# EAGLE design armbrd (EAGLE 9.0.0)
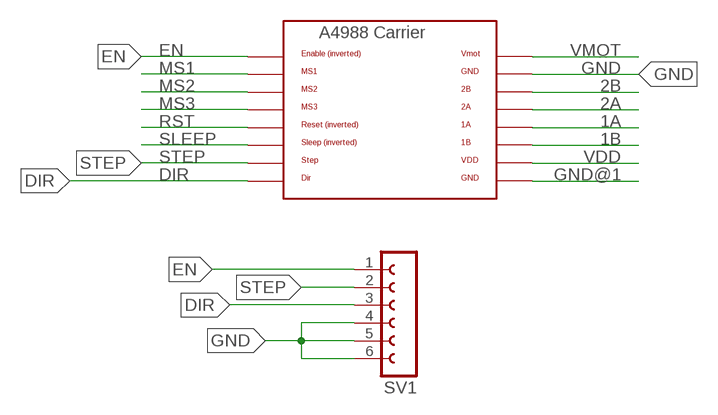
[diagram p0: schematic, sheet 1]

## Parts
SV1  FE06-1  [FE06]
U$1  A4988BREAKOUT  [A4988BREAKOUT]

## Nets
1A: U$1.1A
1B: U$1.1B
2A: U$1.2A
2B: U$1.2B
DIR: SV1.3 U$1.DIR
EN: SV1.1 U$1.EN
GND: SV1.4 SV1.5 SV1.6 U$1.GND
GND@1: U$1.GND@0(GND)
MS1: U$1.MS1
MS2: U$1.MS2
MS3: U$1.MS3
RST: U$1.RST
SLEEP: U$1.SLP(SLEEP)
STEP: SV1.2 U$1.STEP
VDD: U$1.VDD
VMOT: U$1.VMOT

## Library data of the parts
SV1 = con-lsta:FE06-1: FEMALE HEADER; OC_FARNELL: unknown; OC_NEWARK: unknown
U$1 = RepRapjr:A4988BREAKOUT

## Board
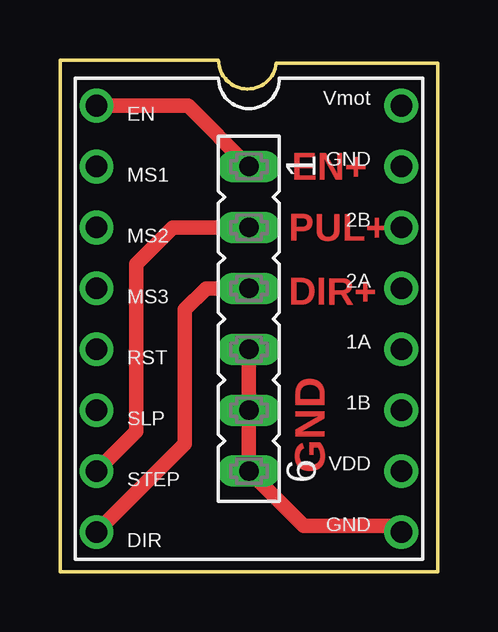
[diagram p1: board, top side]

Size 15.75 x 21.34 mm. Coordinates in mm from the lower left corner, seen from the top.
Outline: 0,21.34 6.6,21.34 arc174 9.02,21.21 15.75,21.21 15.75,0 0,0 0,21.34
Copper layers (1*16): Top 0.035mm / dielectric 1.5mm / Bottom 0.035mm
Design rules "default": minimum track width 6mil, minimum drill 0.35mm, track to track 6mil, track to pad 6mil, pad to pad 6mil, via to via 6mil, smd to smd 6mil, copper to edge 40mil, drill to drill 6mil, minimum pad ring 10mil, minimum via ring 8mil, stop-mask expansion 4mil, vias tented up to drill 0mil, thermal gap 10mil

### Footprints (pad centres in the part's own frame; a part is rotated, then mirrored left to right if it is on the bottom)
FE06 = drill 0.813 long: 1 -6.35,0; 2 -3.81,0; 3 -1.27,0; 4 1.27,0; 5 3.81,0; 6 6.35,0
A4988BREAKOUT = drill 0.9: 1A 8.89,1.27; 1B 11.43,1.27; 2A 6.35,1.27; 2B 3.81,1.27; DIR 16.51,-11.43; EN -1.27,-11.43; GND 16.51,1.27; GND@0 1.27,1.27; MS1 1.27,-11.43; MS2 3.81,-11.43; MS3 6.35,-11.43; RST 8.89,-11.43; SLP 11.43,-11.43; STEP 13.97,-11.43; VDD 13.97,1.27; VMOT -1.27,1.27

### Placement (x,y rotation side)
SV1  7.87,10.54 270 top
U$1  12.95,18.16 270 top

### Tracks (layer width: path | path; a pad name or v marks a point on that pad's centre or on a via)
DIR
  Top 0.61: U$1.DIR 5.21,5.33 5.21,10.92 6.1,11.81 SV1.3
EN
  Top 0.61: U$1.EN 5.33,19.43 SV1.1
GND
  Top 0.61: SV1.4 SV1.5 SV1.6 10.16,1.91 13.72,1.91 13.97,1.65 U$1.GND
STEP
  Top 0.61: U$1.STEP 3.17,5.84 3.17,12.83 4.7,14.35 SV1.2

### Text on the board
Top: EN+ | PUL+ | DIR+ | GND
